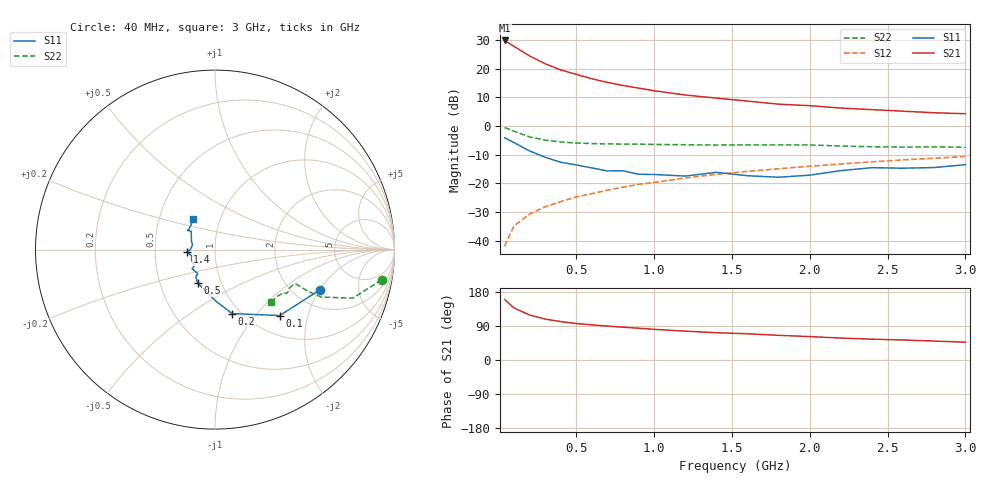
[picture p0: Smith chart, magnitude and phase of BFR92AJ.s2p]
! Filename:  BFR92AJ.S2P  Version:  2.0
! Philips part #: BFR92A  Date: May 1990
! Bias condition: Vce=10V, Ic=20mA
#  MHz  S  MA  R  50
! Freq  S11  S21  S12  S22  !GUM [dB]
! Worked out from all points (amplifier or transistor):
!   21 points, 40 MHz to 3 GHz, reference 50 ohm
!   highest |S21| = 29.9 dB at 40 MHz (marker M1)
!   |S21| within 3 dB of that: start of sweep to 128.4 MHz
!   unconditionally stable (mu >= 1): 680.1 MHz to 758 MHz; 826.7 MHz to 2.388 GHz; 2.554 GHz to 2.609 GHz
!   at 300 MHz: K = 0.83, MSG = 25.0 dB, |S12| = -28.2 dB
!   at 1 GHz: K = 1.03, MAG = 15.0 dB, |S12| = -19.7 dB
!   at 3 GHz: K = 0.97, MSG = 7.5 dB, |S12| = -10.6 dB
!   S11 on the Smith chart (normalised r, x): 40 MHz: 2.73, -2.01; 100 MHz: 1.35, -1.35; 200 MHz: 0.91, -0.75; 500 MHz: 0.77, -0.30; 1.4 GHz: 0.73, -0.02; 3 GHz: 0.74, +0.27
40  0.626 -21.0  31.31 159.5  0.008 79.1  0.944 -10.3
100  0.515 -45.5  24.71 137.6  0.018 71.0  0.814 -19.4
200  0.369 -75.0  16.85 118.7  0.029 69.8  0.648 -24.1
300  0.286 -89.3  12.29 108.0  0.039 70.6  0.57 -24.1
400  0.234 -103.4  9.573 101.5  0.048 72.1  0.529 -23.7
500  0.21 -117.5  8.014 96.2  0.058 72.2  0.507 -23.2
600  0.186 -125.0  6.718 92.7  0.066 73.6  0.495 -23.2
700  0.165 -125.8  5.801 89.6  0.076 75.2  0.488 -23.3
800  0.166 -140.0  5.129 86.5  0.086 75.0  0.486 -23.7
900  0.144 -142.5  4.61 83.9  0.096 76.3  0.484 -24.1
1000  0.143 -156.2  4.152 80.9  0.104 76.1  0.478 -24.2
1200  0.134 -164.4  3.493 76.2  0.124 75.6  0.473 -25.4
1400  0.156 -175.1  3.081 72.0  0.144 74.5  0.467 -27.4
1600  0.136 178.9  2.736 69.2  0.162 74.5  0.47 -28.7
1800  0.128 167.9  2.415 65.1  0.18 74.2  0.47 -30.2
2000  0.139 160.4  2.274 61.8  0.199 73.0  0.468 -31.5
2200  0.167 142.5  2.064 57.8  0.218 73.1  0.449 -32.6
2400  0.188 144.7  1.94 55.0  0.238 71.5  0.436 -36.1
2600  0.184 145.3  1.82 52.8  0.257 70.7  0.43 -39.5
2800  0.189 135.6  1.712 49.9  0.275 70.2  0.434 -42.0
3000  0.212 125.4  1.644 47.0  0.294 68.7  0.426 -42.9
